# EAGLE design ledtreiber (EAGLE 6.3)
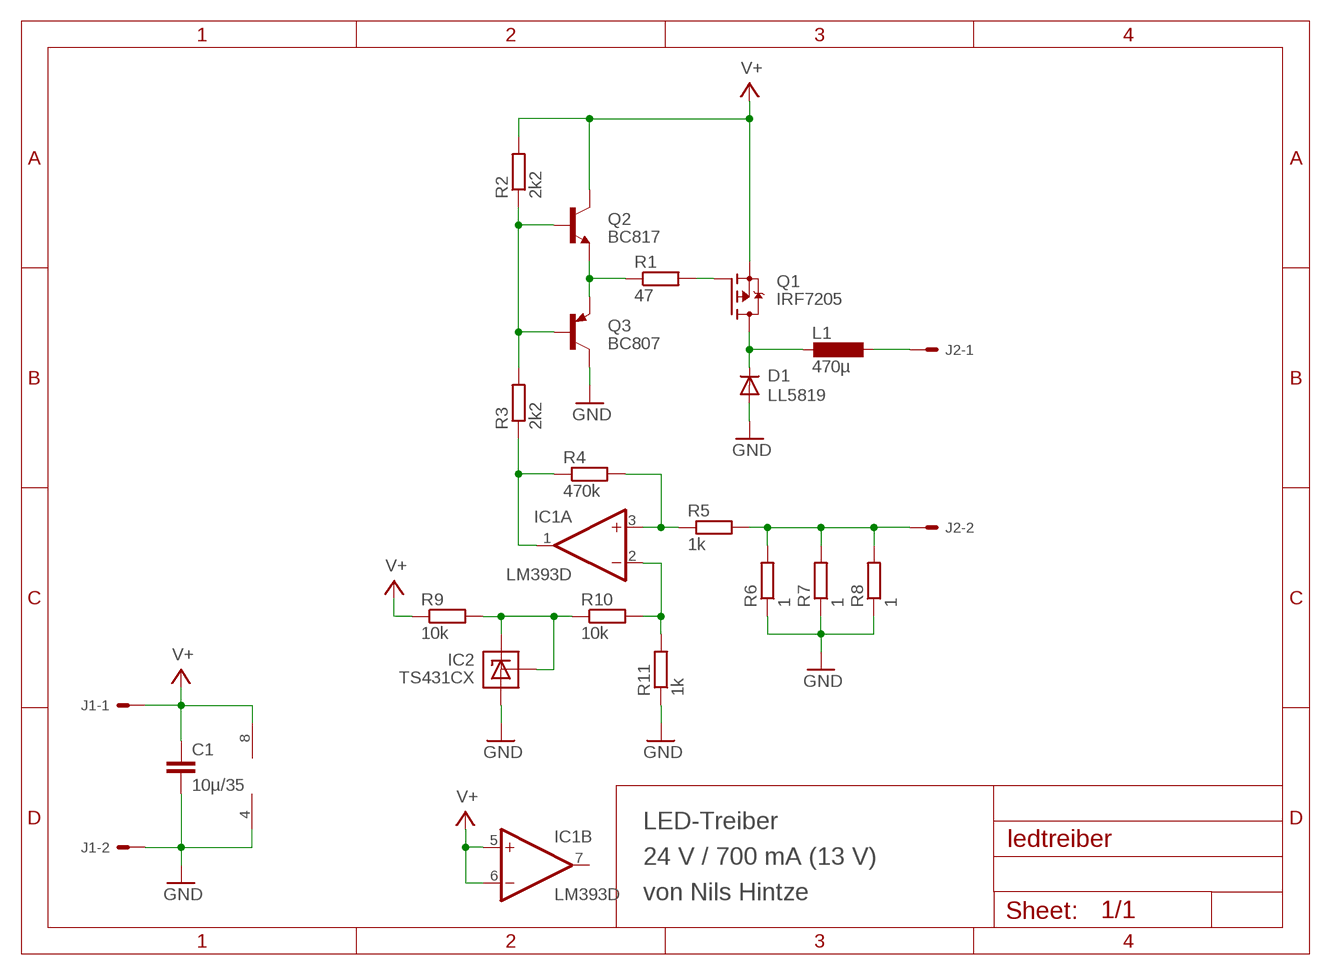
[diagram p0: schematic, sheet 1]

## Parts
C1  10µ/35  C-EUC1210  [C1210]
D1  LL5819  DIODE-MELF-MLL41  [MELF-MLL41]
IC1  LM393D  [SO08]
IC2  TS431CX  431-SOT23  [SOT23]
J1  22-27-2021-02  [6410-02]
J2  22-27-2021-02  [6410-02]
L1  470µ  LPISR_LARGEPADS  [PISR_LARGEPADS]
Q1  IRF7205  [SO08]
Q2  BC817  [SOT23-BEC_GROSSER_ABSTAND]
Q3  BC807  [SOT23-BEC_GROSSER_ABSTAND]
R1  47  R-EU_R0805  [R0805]
R2  2k2  R-EU_R0805  [R0805]
R3  2k2  R-EU_R0805  [R0805]
R4  470k  R-EU_R0805  [R0805]
R5  1k  R-EU_R0805  [R0805]
R6  1  R-EU_R0805  [R0805]
R7  1  R-EU_R0805  [R0805]
R8  1  R-EU_R0805  [R0805]
R9  10k  R-EU_R0805  [R0805]
R10  10k  R-EU_R0805  [R0805]
R11  1k  R-EU_R0805  [R0805]

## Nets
GND: C1.2 D1.A IC1.4(P:V-) IC2.3(A) J1.2 Q3.C R6.1 R7.1 R8.1 R11.1
N$1: Q2.E Q3.E R1.1
N$2: Q1.4(G) R1.2
N$3: J2.1 L1.1
N$4: J2.2 R5.2 R6.2 R7.2 R8.2
N$5: Q2.B Q3.B R2.1 R3.2
N$6: D1.C L1.2 Q1.5(D) Q1.6(D) Q1.7(D) Q1.8(D)
N$7: IC1.1(A:OUT) R3.1 R4.1
N$8: IC1.3(A:+IN) R4.2 R5.1
N$9: IC2.1(REF) IC2.2(C) R9.2 R10.1
N$11: IC1.2(A:-IN) R10.2 R11.2
V+: C1.1 IC1.5(B:+IN) IC1.6(B:-IN) IC1.8(P:V+) J1.1 Q1.1(S) Q1.2(S) Q1.3(S) Q2.C R2.2 R9.1
Unconnected: IC1.7(B:OUT)

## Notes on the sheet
- LED-Treiber
- 24 V / 700 mA (13 V)
- von Nils Hintze

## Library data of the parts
C1 = rcl:C-EU: CAPACITOR, European symbol
D1 = diode:DIODE-: DIODE
IC1 = linear:LM393: COMPARATOR
IC2 = nh-ref-431:431
J1 J2 = con-molex:22-?-02: CONNECTOR; OC_FARNELL: unknown; OC_NEWARK: unknown
L1 = nh-inductor-pisr:L
Q1 = nh-irf7205:IRF7205
Q2 = nh_transistor-npn:BC817*: NPN Transistor
Q3 = nh_transistor-pnp:BC807*: PNP Transistror
R1-R11 = rcl:R-EU_: RESISTOR, European symbol

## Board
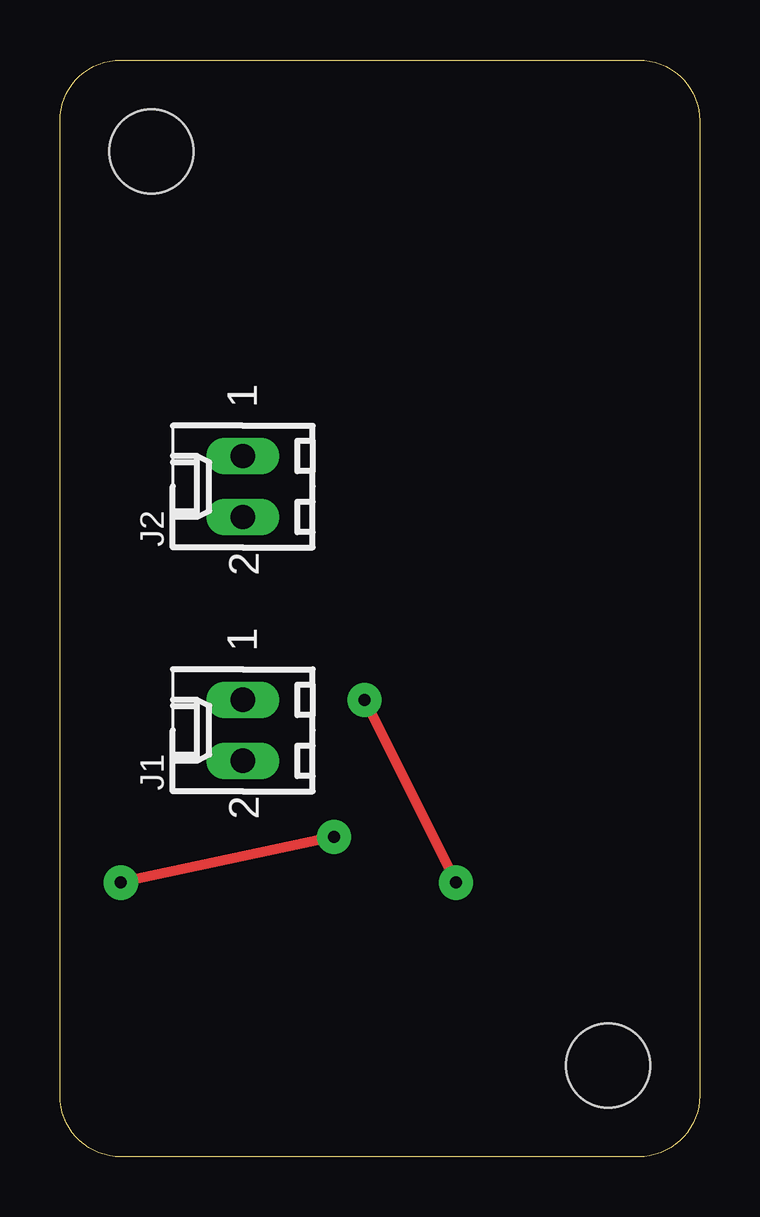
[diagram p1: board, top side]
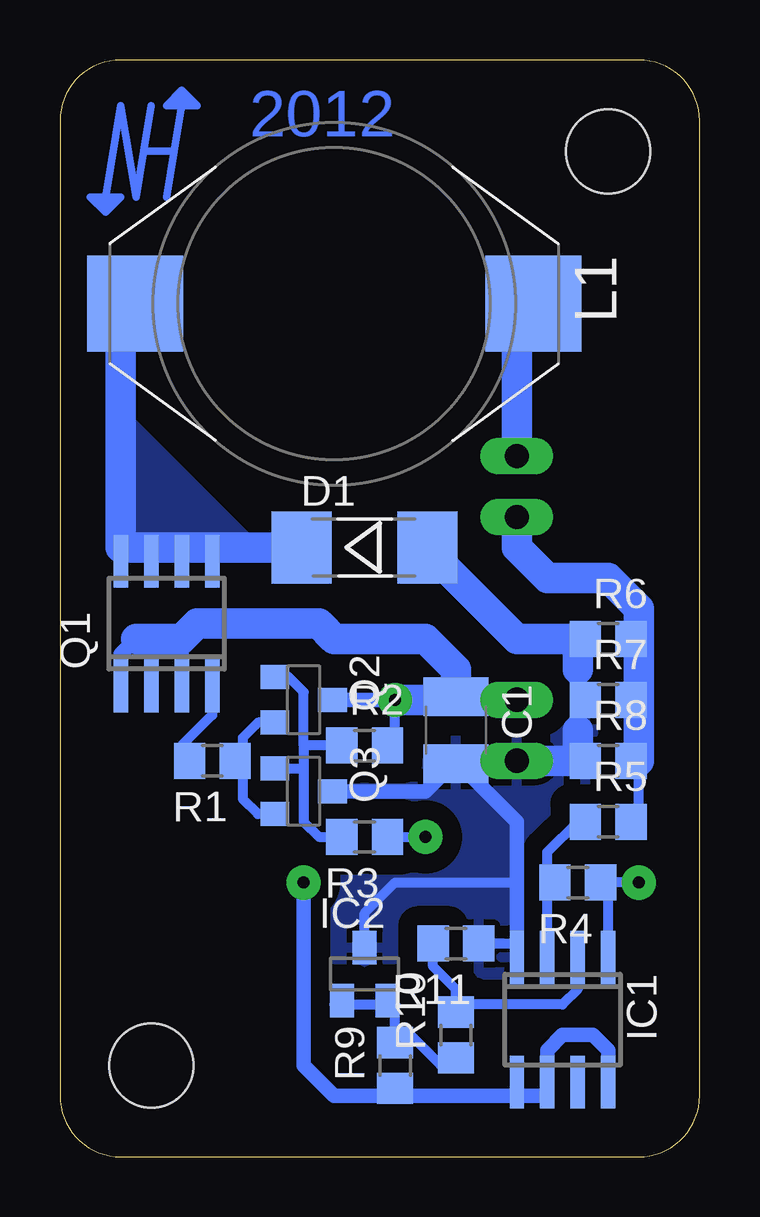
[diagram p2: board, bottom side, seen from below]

Size 26.67 x 45.72 mm. Coordinates in mm from the lower left corner, seen from the top.
Outline: 2.54,0 arc-90 0,2.54 0,43.18 arc-90 2.54,45.72 24.13,45.72 arc-90 26.67,43.18 26.67,2.54 arc-90 24.13,0 2.54,0
Copper layers (1*16): Top 0.035mm / dielectric 1.5mm / Bottom 0.035mm
Design rules "default": minimum track width 10mil, minimum drill 24mil, track to track 8mil, track to pad 8mil, pad to pad 8mil, via to via 8mil, smd to smd 8mil, copper to edge 40mil, drill to drill 8mil, minimum pad ring 10mil, minimum via ring 8mil, stop-mask expansion 4mil, vias tented up to drill 0mil, thermal gap 10mil
Holes 3.5 mm at 22.86,3.81 3.81,41.91
bRestrict: area 0,38.1 to 7.6,45.7; area 19.1,0 to 26.7,7.6

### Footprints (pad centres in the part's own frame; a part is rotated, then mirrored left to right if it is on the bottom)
C1210 = smd 1.6 x 2.7: 1 -1.4,0; 2 1.4,0
MELF-MLL41 = smd 2.5 x 3: A 2.625,0; C -2.625,0
SO08 = smd 0.6 x 2.2: 1 -1.905,-2.6; 2 -0.635,-2.6; 3 0.635,-2.6; 4 1.905,-2.6; 5 1.905,2.6; 6 0.635,2.6; 7 -0.635,2.6; 8 -1.905,2.6
SOT23 = smd 1 x 1.4: 1 -0.95,-1.1; 2 0.95,-1.1; 3 0,1.1
6410-02 = drill 1.016 long: 1 1.27,0; 2 -1.27,0
PISR_LARGEPADS = smd 4 x 4: 1 0,8.3; 2 0,-8.3
SOT23-BEC_GROSSER_ABSTAND = smd 1 x 1.2: B -0.95,-1.2; C 0,1.2; E 0.95,-1.2
R0805 = smd 1.3 x 1.5: 1 -0.95,0; 2 0.95,0

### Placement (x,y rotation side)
C1  10.16,17.78 270 bottom
D1  13.97,25.4 0 bottom
IC1  5.71,5.71 180 bottom
IC2  13.97,7.62 0 bottom
J1  7.62,17.78 90 top
J2  7.62,27.94 90 top
L1  15.24,35.56 270 bottom
Q1  22.23,22.23 0 bottom
Q2  16.51,19.05 270 bottom
Q3  16.51,15.24 270 bottom
R1  20.32,16.51 180 bottom
R2  13.97,17.14 0 bottom
R3  13.97,13.34 180 bottom
R4  5.08,11.43 180 bottom
R5  3.81,13.97 0 bottom
R6  3.81,21.59 0 bottom
R7  3.81,19.05 0 bottom
R8  3.81,16.51 0 bottom
R9  12.7,3.81 90 bottom
R10  10.16,5.08 90 bottom
R11  10.16,8.89 180 bottom

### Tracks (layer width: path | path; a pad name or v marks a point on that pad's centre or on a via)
GND
  Bottom 0.406: R11.1 7.62,8.89 | IC2.3 13.97,10.16 12.7,11.43 7.62,11.43
  Bottom 0.61: 5.08,20.32 5.08,19.05 | 5.08,19.05 5.08,17.78 | R7.1 5.08,19.05 | Q3.C 11.43,15.24 10.16,16.51 7.62,13.97 7.62,11.43 7.62,8.89 IC1.4
  Bottom 1.27: 5.08,21.59 5.08,20.32 | 5.08,17.78 5.08,16.51 | R6.1 5.08,21.59 | R8.1 5.08,16.51 | C1.2 10.16,16.51 J1.2 5.08,16.51 | 5.08,21.59 7.62,21.59 11.43,25.4 D1.A
  pour Bottom (isolate 0.813): 26.67,0 0,0 0,19.05 26.67,19.05
N$1
  Bottom 0.406: Q3.E 18.41,14.29 19.05,14.92 19.05,16.51 | Q2.E 18.41,18.1 19.05,17.46 19.05,16.51 | R1.1 19.05,16.51
N$2
  Bottom 0.406: Q1.4 20.32,18.41 21.59,17.14 R1.2
N$3
  Bottom 1.27: L1.1 7.62,35.56 J2.1
N$4
  Bottom 0.406: R5.2 2.54,13.97 2.54,16.51
  Bottom 1.27: R8.2 2.54,16.51 2.54,19.05 | 2.54,19.05 2.54,21.59 | 2.54,21.59 2.54,22.86 3.81,24.13 6.35,24.13 7.62,25.4 J2.2 | R6.2 2.54,21.59 | R7.2 2.54,19.05
N$5
  Bottom 0.406: 16.51,17.14 16.51,19.37 17.14,20 Q2.B | 16.51,17.14 16.51,16.19 | 16.51,16.19 16.51,13.97 15.88,13.34 R3.2 | R2.1 16.51,17.14 | Q3.B 16.51,16.19
N$6
  Bottom 0.61: Q1.5 20.32,25.4 | Q1.6 21.59,25.4 | Q1.7 22.86,25.4 | Q1.8 24.13,25.4
  Bottom 1.27: L1.2 24.13,35.56 24.13,25.4 22.86,25.4 21.59,25.4 20.32,25.4 D1.C
  pour Bottom: 24.13,25.4 19.05,25.4 24.13,30.48
N$7  (via drill 0.5 pad 1.42)
  Top 0.406: v11.43,13.34 v2.54,11.43
  Bottom 0.406: R3.1 v11.43,13.34 | v2.54,11.43 3.81,11.43 | 3.81,11.43 R4.1 | IC1.1 3.81,11.43
N$8
  Bottom 0.406: IC1.3 6.35,11.43 | 6.35,11.43 6.35,12.7 5.08,13.97 R5.1 | R4.2 6.35,11.43
N$9
  Bottom 0.406: R10.1 10.16,3.81 10.79,3.81 12.06,5.08 12.7,5.08 | R9.2 12.7,5.08 | 12.7,5.08 12.7,6.35 12.85,6.35 | IC2.1 15.07,6.52 15.24,6.35 12.85,6.35 | 12.85,6.35 IC2.2
N$11
  Bottom 0.406: IC1.2 5.08,6.99 5.71,6.35 10.16,6.35 | 10.16,6.35 10.16,6.99 11.11,7.93 R11.2 | R10.2 10.16,6.35
N$25
  Bottom 0.305: 24.77,40.01 24.13,43.81 23.5,40.01 23.18,41.91 | 23.18,41.91 22.86,43.81 | 21.91,41.91 23.18,41.91 | 21.91,41.91 21.59,43.81 | 22.23,40.01 21.91,41.91 | 24.77,40.01 25.4,40.01 | 25.4,40.01 24.77,39.37 | 24.13,40.01 24.77,39.37 | 24.77,40.01 24.13,40.01 | 21.59,43.81 22.23,43.81 | 22.23,43.81 21.59,44.45 | 20.95,43.81 21.59,44.45 | 21.59,43.81 20.95,43.81 | 21.59,43.81 21.59,44.13 | 21.59,44.13 21.59,44.45 | 24.77,40.01 24.77,39.69 | 24.77,39.69 24.77,39.37 | 20.95,43.81 21.59,44.13 | 22.23,43.81 21.59,44.13 | 24.13,40.01 24.77,39.69 | 25.4,40.01 24.77,39.69
V+  (via drill 0.5 pad 1.42)
  Top 0.406: v12.7,19.05 v16.51,11.43
  Bottom 0.406: R2.2 12.7,17.14 v12.7,19.05 | IC1.6 6.35,2.54 | R9.1 12.7,2.54
  Bottom 0.61: Q1.1 24.13,20.95 23.5,21.59 | Q1.2 22.86,21.59 | Q1.3 21.59,21.59 | Q2.C v12.7,19.05 | 3.81,2.54 IC1.8 3.81,4.45 4.45,5.08 5.71,5.08 6.35,4.45 IC1.6 | 7.62,2.54 6.35,2.54 | IC1.5 7.62,2.54 | 7.62,2.54 12.7,2.54 15.24,2.54 16.51,3.81 v16.51,11.43
  Bottom 1.27: 23.5,21.59 22.86,21.59 21.59,21.59 20.95,22.23 15.88,22.23 15.24,21.59 11.43,21.59 10.16,20.32 C1.1 10.16,19.05 | v12.7,19.05 10.16,19.05 | 10.16,19.05 J1.1

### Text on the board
Bottom: 2012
